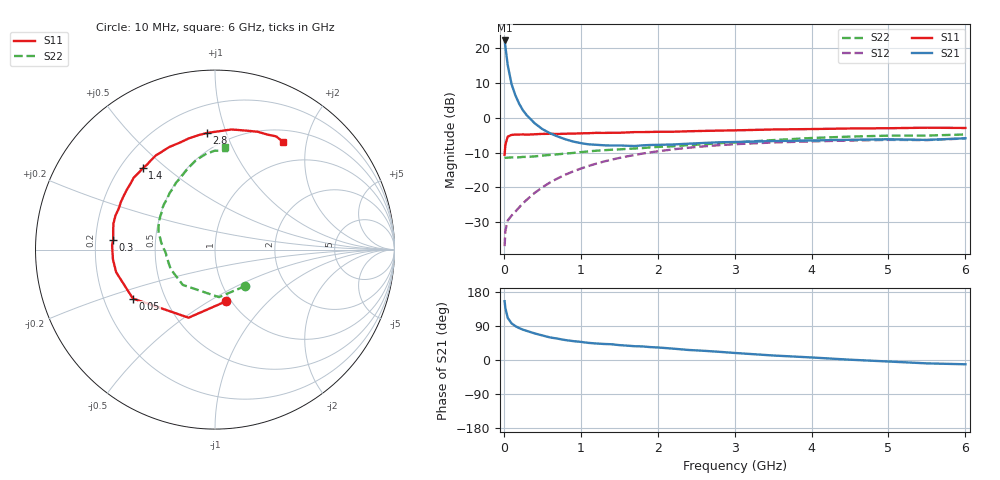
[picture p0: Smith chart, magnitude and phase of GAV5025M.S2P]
! Infineon Technologies  Discrete & RF Semiconductors
! BF775
! Si NPN RF Bipolar Junction Transistor in SOT23
! VCE = 0.5 V  IC = 25 mA
! Common Emitter S-Parameters:  May  1996
# GHz  S  MA  R  50
!  f  S11  S21  S12  S22
! GHz  MAG  ANG  MAG  ANG  MAG  ANG  MAG  ANG
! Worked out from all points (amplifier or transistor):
!   36 points, 10 MHz to 6 GHz, reference 50 ohm
!   highest |S21| = 22.1 dB at 10 MHz (marker M1)
!   |S21| within 3 dB of that: start of sweep to 27.29 MHz
!   unconditionally stable (mu >= 1): start of sweep to end of sweep
!   at 250 MHz: K = 4.28, MAG = 4.0 dB, |S12| = -24.6 dB
!   at 1.4 GHz: K = 3.06, MAG = -5.7 dB, |S12| = -12.1 dB
!   at 6 GHz: K = 1.17, MAG = -2.5 dB, |S12| = -6.0 dB
!   S11 on the Smith chart (normalised r, x): 10 MHz: 0.95, -0.60; 50 MHz: 0.33, -0.25; 300 MHz: 0.27, +0.04; 1.4 GHz: 0.29, +0.42; 2.8 GHz: 0.38, +0.86; 6 GHz: 0.67, +1.61
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0.01  0.2941 -77.5  12.73 155.2  0.0144 60.2  0.2639 -50.2
0.02  0.4069 -111.2  10.45 137.1  0.0239 49.6  0.2658 -85.2
0.05  0.5325 -149.2  5.685 111.4  0.0335 37.1  0.2664 -132.5
0.1  0.565 -167.1  3.029 96.8  0.0394 37.9  0.2695 -156.3
0.15  0.5712 -174.5  2.082 89.4  0.045 42.9  0.2692 -164.5
0.2  0.5716 -179.1  1.573 84.1  0.0519 48.3  0.2699 -169.3
0.25  0.5737 177.4  1.264 79.9  0.0592 51.7  0.2737 -172.5
0.3  0.5696 174.6  1.074 76.7  0.0669 54.9  0.2733 -174.5
0.4  0.577 169.5  0.831 70.2  0.0833 58.4  0.278 -177.9
0.5  0.5842 165.6  0.685 64.8  0.1002 60.0  0.2856 179.0
0.6  0.586 161.2  0.597 59.6  0.1176 60.5  0.2922 176.4
0.8  0.5876 153.2  0.489 52.6  0.1522 59.3  0.3052 171.3
1.1  0.5977 141.8  0.414 45.2  0.2027 55.6  0.3282 163.0
1.4  0.6057 131.6  0.398 41.6  0.2495 50.4  0.3464 154.6
1.7  0.62 121.9  0.392 36.4  0.2911 45.2  0.3608 146.1
2.2  0.6273 108.3  0.412 30.0  0.3507 35.9  0.3881 133.8
2.8  0.6512 93.9  0.443 21.6  0.4028 25.5  0.4306 120.4
3.5  0.6757 82.1  0.461 11.9  0.44 14.7  0.4758 108.7
4.5  0.6984 70.1  0.481 0.8  0.4692 2.5  0.5344 95.6
5  0.7041 65.5  0.489 -4.0  0.4795 -2.8  0.5513 90.1
5.5  0.7169 61.6  0.479 -8.9  0.4762 -8.1  0.5525 82.9
6  0.71 57.6  0.506 -11.3  0.5023 -11.4  0.5733 84.5
